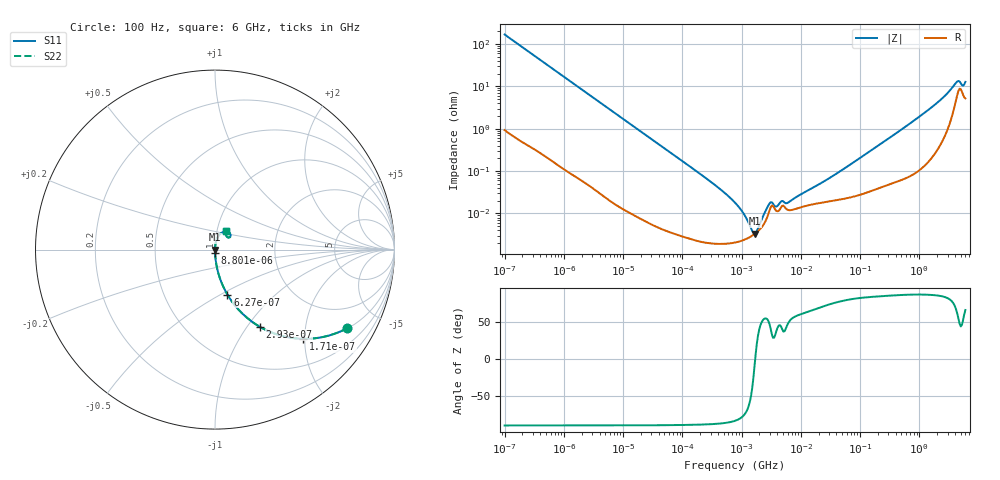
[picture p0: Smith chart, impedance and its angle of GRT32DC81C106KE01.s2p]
!Murata Part Number: GRT32DC81C106KE01
!These Parameters are Measured in Series Mode Connection
!Data Generated on Jun 19, 2026
!  o--ll--o
!Port1  Port2
!  o------o
!Operation Temp=25[degC], DC Bias Voltage=0[V]
!Freq. Start=100[Hz] Stop=6[GHz] 401[Steps]
# Hz S RI R 50
!Freq.(Hz) S11(Real) S11(Imag) S21(Real) S21(Imag) S12(Real) S12(Imag) S22(Real) S22(Imag)
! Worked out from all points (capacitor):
!   401 points, 100 Hz to 6 GHz, reference 50 ohm
!   read as one part in series: C = 9.45 uF near 109 Hz
!   lowest |Z| = 3.3 mohm at 1.658 MHz (marker M1)
!   series resonance near 1.699 MHz, so ESL is about 930 pH
!   S11 on the Smith chart (normalised r, x): 100 Hz: 1.02, -3.36; 171 Hz: 1.01, -1.97; 293 Hz: 1.01, -1.15; 627 Hz: 1.00, -0.54; 8.801 kHz: 1.00, -0.04; 6 GHz: 1.10, +0.23
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100  0.7378 -0.4371  0.2622 0.4371  0.2622 0.4371  0.7378 -0.4371
171  0.4923 -0.4972  0.5077 0.4972  0.5077 0.4972  0.4923 -0.4972
293  0.2507 -0.4304  0.7493 0.4304  0.7493 0.4304  0.2507 -0.4304
627  0.0694 -0.251  0.9306 0.251  0.9306 0.251  0.0694 -0.251
2008  0.00771 -0.084  0.9923 0.084  0.9923 0.084  0.00771 -0.084
8801  0.000518 -0.0194  0.9995 0.0194  0.9995 0.0194  0.000518 -0.0194
40335  6.36e-05 -0.00427  0.9999 0.00427  0.9999 0.00427  6.36e-05 -0.00427
330837  1.96e-05 -0.000506  1 0.000506  1 0.000506  1.96e-05 -0.000506
774597  2.06e-05 -0.000179  1 0.000179  1 0.000179  2.06e-05 -0.000179
1108252  2.38e-05 -9.1e-05  1 9.1e-05  1 9.1e-05  2.38e-05 -9.1e-05
1658239  3.26e-05 -5.1e-06  1 5.1e-06  1 5.1e-06  3.26e-05 -5.1e-06
2268635  5.06e-05 6.47e-05  0.9999 -6.47e-05  0.9999 -6.47e-05  5.06e-05 6.47e-05
3103719  0.00014 0.000119  0.9999 -0.000119  0.9999 -0.000119  0.00014 0.000119
3882480  0.000114 8.94e-05  0.9999 -8.94e-05  0.9999 -8.94e-05  0.000114 8.94e-05
4856642  0.000151 0.000127  0.9998 -0.000127  0.9998 -0.000127  0.000151 0.000127
6075234  0.000121 0.000133  0.9999 -0.000133  0.9999 -0.000133  0.000121 0.000133
1.555665e7  0.000163 0.000361  0.9998 -0.000361  0.9998 -0.000361  0.000163 0.000361
4.556224e7  0.000213 0.000956  0.9998 -0.000956  0.9998 -0.000956  0.000213 0.000956
3.124326e8  0.000524 0.00603  0.9995 -0.00603  0.9995 -0.00603  0.000524 0.00603
1.791126e9  0.00374 0.0357  0.9963 -0.0357  0.9963 -0.0357  0.00374 0.0357
4.193612e9  0.0577 0.1013  0.9423 -0.1013  0.9423 -0.1013  0.0577 0.1013
6e9  0.0609 0.1041  0.9391 -0.1041  0.9391 -0.1041  0.0609 0.1041
